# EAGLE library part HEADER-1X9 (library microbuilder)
PIN HEADER
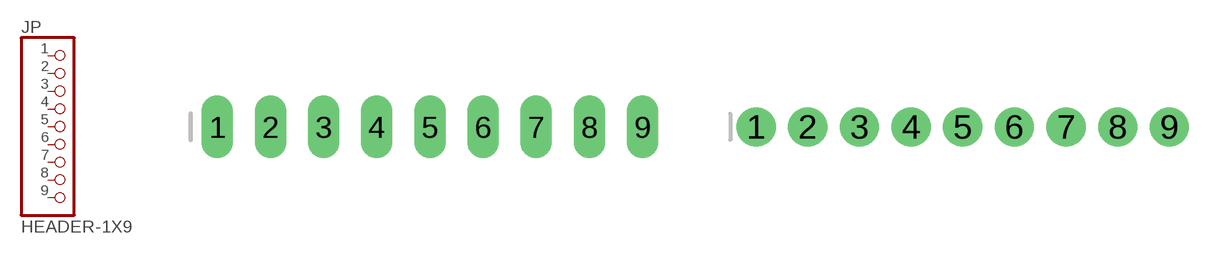
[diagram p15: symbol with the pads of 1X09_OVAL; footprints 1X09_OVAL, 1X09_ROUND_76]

Designator prefix JP

## HEADER-1X9  [1X09_OVAL]
1  1  pas
2  2  pas
3  3  pas
4  4  pas
5  5  pas
6  6  pas
7  7  pas
8  8  pas
9  9  pas

## HEADER-1X976MIL  [1X09_ROUND_76]
Pads as for 1X09_OVAL

## HEADER-1X970MIL  [1X09_ROUND_70]
Pads as for 1X09_OVAL

## Footprint 1X09_OVAL (pad centres in mm)
PIN HEADER
drill 1 long: 1 -10.16,0; 2 -7.62,0; 3 -5.08,0; 4 -2.54,0; 5 0,0; 6 2.54,0; 7 5.08,0; 8 7.62,0; 9 10.16,0

## Footprint 1X09_ROUND_76 (pad centres in mm)
drill 1 pad 1.93: 1 -10.16,0; 2 -7.62,0; 3 -5.08,0; 4 -2.54,0; 5 0,0; 6 2.54,0; 7 5.08,0; 8 7.62,0; 9 10.16,0

## Footprint 1X09_ROUND_70 (pad centres in mm)
drill 1 pad 1.778: 1 -10.16,0; 2 -7.62,0; 3 -5.08,0; 4 -2.54,0; 5 0,0; 6 2.54,0; 7 5.08,0; 8 7.62,0; 9 10.16,0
